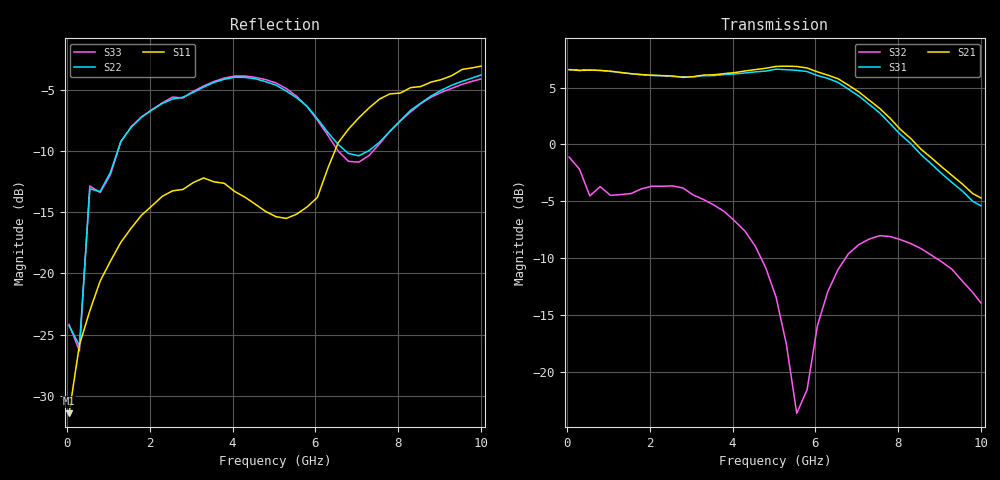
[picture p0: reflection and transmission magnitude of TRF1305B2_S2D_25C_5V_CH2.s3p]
! Created Wed Jul  2 22:03:19 2025
# hz S ma R 50
! 3 Port Network Data from SP1.SP block
! PORT[1] = INP
! PORT[2]= OUTM
! PORT[3] = OUTP
! freq  magS11  angS11  magS12  angS12  magS13  angS13
!  magS21  angS21
!  magS22  angS22  magS23  angS23
!  magS31  angS31  magS32  angS32
!  magS33  angS33
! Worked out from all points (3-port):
!   41 points, 50 MHz to 10 GHz, reference 50 ohm
!   strongest paths, dB at 50 MHz, 2.55 GHz, 5.05 GHz, 7.55 GHz, 10 GHz:
!     S21: 6.6, 6.0, 6.9, 3.2, -4.7
!     S31: 6.6, 6.0, 6.6, 2.8, -5.4
!     S32: -1.1, -3.6, -13.4, -8.0, -13.9
!   lowest |S11| = -31.4 dB at 50 MHz (marker M1), VSWR 1.06, Z = 47.5 - j0.631 ohm
!   |S11| at or under -10 dB: start of sweep to 6.471 GHz
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5e7  0.02684 -165.7  0.002127 -27.1  0.004311 -149.4
     2.131 177.9  0.06108 25.3  0.8803 0.5
     2.134 -2.2  0.8802 0.3  0.06189 24.0
3e8  0.05108 -130.3  0.004104 26.8  0.001369 -138.8
     2.113 168.7  0.05074 153.4  0.7771 -6.6
     2.127 -11.5  0.7792 -6.4  0.04822 151.9
5.5e8  0.07038 -123.9  0.01472 65.1  0.009792 89.8
       2.123 159.4  0.2215 169.4  0.6046 -15.1
       2.123 -20.3  0.594 -15.2  0.2277 168.6
2.55e9  0.2175 -139.2  0.02779 25.1  0.008219 -79.1
        1.998 87.8  0.5154 59.2  0.662 -27.7
        1.991 -91.2  0.6574 -26.8  0.5252 59.3
3.8e9  0.2334 -155.5  0.04709 21.0  0.01404 174.0
       2.048 44.7  0.6208 33.6  0.5078 -51.3
       2.028 -134.9  0.5071 -51.2  0.6279 33.5
5.05e9  0.1705 -156.5  0.09423 -16.9  0.008389 92.7
        2.203 -4.9  0.5877 6.6  0.207 -80.5
        2.142 175.7  0.2135 -75.7  0.5999 6.0
5.55e9  0.1748 -149.5  0.1099 -39.7  0.004653 131.4
        2.202 -28.4  0.5213 -0.9  0.04775 -37.9
        2.118 152.2  0.06583 -46.0  0.5289 -3.3
6.55e9  0.3413 -143.7  0.1168 -77.6  0.01403 90.2
        1.943 -76.0  0.3363 -1.3  0.2999 19.6
        1.872 104.0  0.2824 18.6  0.3162 -4.8
7.8e9  0.5412 -175.3  0.1026 -123.5  0.01367 44.0
       1.307 -131.0  0.3801 27.1  0.3936 -12.6
       1.238 48.1  0.3941 -11.7  0.38 28.9
1e10  0.7022 149.3  0.07139 -174.1  0.00926 13.0
      0.5824 164.4  0.646 9.1  0.2115 -34.8
      0.5378 -19.0  0.2012 -36.5  0.6222 10.4
